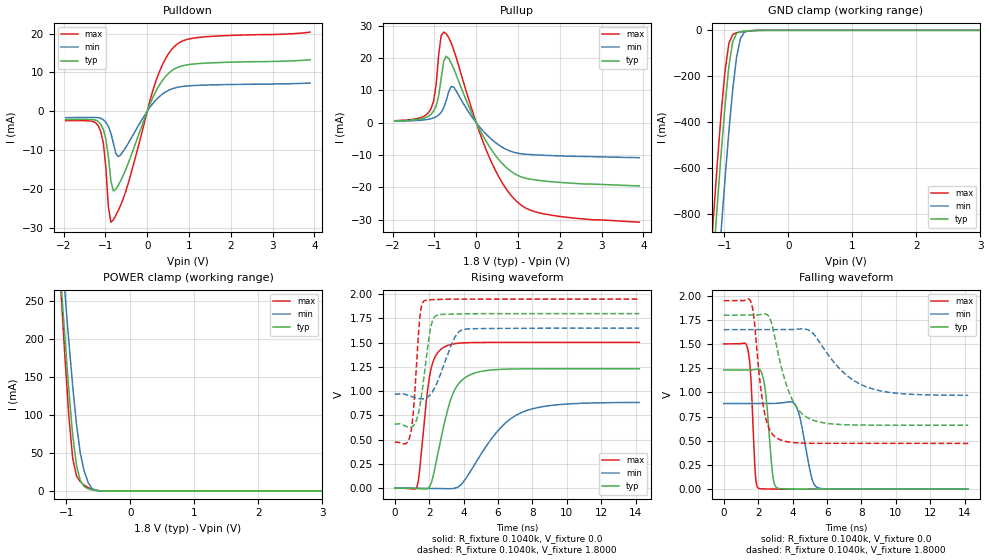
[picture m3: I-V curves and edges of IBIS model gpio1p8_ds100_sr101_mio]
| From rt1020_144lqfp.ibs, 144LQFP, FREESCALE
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[Model] gpio1p8_ds100_sr101_mio
|   Model gpio1p8_ds100_sr101_mio
| This model was characterised for following simulation conditions:
| External (pad) voltage:
|   - Typ: 1.8V,   - Min: 1.65V,   - Max: 1.95V
| Library cells for typ/min/max conditions are connected as defined below:
|  pad - External Pad
|  ipp_do - Core Input
|  ipp_obe - Output Buffer Enable
|  esd_boost - ovdd
|  ipp_dse0 - vssi
|  ipp_dse1 - vssi
|  ipp_dse2 - vddi
|  ipp_fsel0 - vddi
|  ipp_fsel1 - vssi
|  ipp_ina - ipp_ina
|  ipp_ind - ipp_ind
|  ipp_pwr_stable - vddi
|  ipp_sre - vddi
|  ovdd - ovdd
|  ovss - ovss
|  vddi - vddi
|  vssi - vssi
| All other pins connected to ground
Model_type I/O
Polarity   Non-Inverting
Enable   Active-High
Vinl =   0.5400V
Vinh =   1.2600V
Vmeas =  0.9000V
Cref =   0.0F
Rref =   0.1040k
Vref =   0.9000V
C_comp   1.2573pF   1.2208pF   1.3054pF
|C_comp_pullup   0.6439pF   0.6609pF   0.6284pF
|C_comp_pulldown   0.5473pF   0.5786pF   0.5258pF
[Model Spec]
| variable   typ   min   max
Vinh   1.2600V   1.1550V   1.3650V
Vinl   0.5400V   0.4950V   0.5850V
S_overshoot_high   1.8000V   1.6500V   1.9500V
S_overshoot_low   0.0V   0.0V   0.0V
Vmeas   0.9000V   0.8250V   0.9750V
Vref   0.9000V   0.8250V   0.9750V
Cref   0.0F   0.0F   0.0F
Rref   0.1040k   0.1040k   0.1040k
[Temperature Range]   25.0000   0.1050k   -20.0000
[Voltage Range]   1.8000V   1.6500V   1.9500V
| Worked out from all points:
|   slope of the pulldown table from 0 to 0.27 V, typ, clamps not added: 42.3 ohm
|   slope of the pullup table from 0 to 0.27 V, typ, clamps not added: 41.8 ohm
|   GND clamp passes 1 mA (typ) near -0.55 V on its own axis
|   POWER clamp passes 1 mA (typ) near -0.58 V on its own axis
|   rising waveform, R_fixture 0.1040k, V_fixture 0.0: 20-80 % time 1.03ns typ, 2.26ns min, 565ps max; typ from 0 V to 1.23 V
|   rising waveform, R_fixture 0.1040k, V_fixture 1.8000: 20-80 % time 506ps typ, 874ps min, 333ps max; typ from 0.661 V to 1.8 V
|   falling waveform, R_fixture 0.1040k, V_fixture 0.0: 20-80 % time 346ps typ, 561ps min, 230ps max; typ from 1.23 V to 0 V
|   falling waveform, R_fixture 0.1040k, V_fixture 1.8000: 20-80 % time 1.12ns typ, 2.13ns min, 573ps max; typ from 1.8 V to 0.661 V
[Pulldown]
|Voltage   I(typ)   I(min)   I(max)
-1.95V    -2.116mA   -1.648mA   -2.433mA
-1.17V    -2.655mA   -1.64mA    -3.771mA
-1.05V    -4.712mA   -2.199mA   -8.241mA
-990mV    -7.134mA   -2.853mA   -14.49mA
-930mV    -11.63mA   -3.901mA   -24.57mA
-870mV    -17.89mA   -5.605mA   -28.55mA
-810mV    -20.51mA   -8.198mA   -27.94mA
-690mV    -18.99mA   -11.69mA   -25.49mA
210mV     5.219mA    2.926mA    7.83mA
630mV     10.75mA    5.914mA    16.46mA
1.23V     12.27mA    6.677mA    19.01mA
3.9V      13.26mA    7.28mA     20.38mA
[Pullup]
|Voltage   I(typ)   I(min)   I(max)
-1.95V    560uA      440uA      630uA
-1.08V    2.65mA     1.257mA    4.43mA
-960mV    5.224mA    1.847mA    11.81mA
-900mV    8.315mA    2.377mA    20.88mA
-840mV    13.72mA    3.206mA    26.97mA
-780mV    19.01mA    4.561mA    28.05mA
-720mV    20.6mA     6.748mA    27.55mA
-540mV    16.77mA    11mA       22.63mA
240mV     -5.825mA   -3.571mA   -8.452mA
960mV     -16.07mA   -9.337mA   -24.24mA
1.74V     -18.17mA   -10.13mA   -28.48mA
3.9V      -19.55mA   -10.81mA   -30.77mA
[GND_clamp]
|Voltage   I(typ)   I(min)   I(max)
-1.95V    -4.191A    -4.477A    -4.042A
-1.23V    -1.234A    -1.577A    -1.052A
-1.17V    -993.2mA   -1.338A    -811.1mA
-1.11V    -758.1mA   -1.102A    -578.5mA
-1.05V    -533.7mA   -870.8mA   -361.6mA
-990mV    -328mA     -648.8mA   -176.9mA
-930mV    -157.5mA   -441.8mA   -57.56mA
-870mV    -50.13mA   -259.5mA   -18.17mA
-810mV    -13.28mA   -118mA     -10.41mA
-750mV    -5.921mA   -36.52mA   -7.502mA
-630mV    -2.275mA   -2.653mA   -3.283mA
3.9V      0A         0A         0A
[POWER_clamp]
|Voltage   I(typ)   I(min)   I(max)
-1.95V    1.356A     1.328A     1.514A
-1.08V    270.6mA    322.7mA    256.8mA
-1.02V    199mA      258.1mA    173mA
-960mV    131.2mA    195.7mA    97.36mA
-900mV    72.67mA    137.2mA    42.48mA
-840mV    32.99mA    86.34mA    19.5mA
-780mV    13.32mA    48.87mA    11.87mA
-720mV    5.671mA    25.66mA    7.515mA
-660mV    2.793mA    11.19mA    4.477mA
-600mV    1.289mA    3.449mA    2.334mA
-480mV    122.1uA    182.3uA    260.9uA
3.9V      0A         0A         0A
[Ramp]
| variable   typ   min   max
dV/dt_r  0.7391/1.0298n   0.5307/2.2596n   0.9019/0.5652n
dV/dt_f  0.6833/1.1203n   0.4075/2.1341n   0.8860/0.5735n
R_load = 0.1040k
[Rising Waveform]
R_fixture= 0.1040k
V_fixture= 0.0
V_fixture_min= 0.0
V_fixture_max= 0.0
|time   V(typ)   V(min)   V(max)
0s        580.6pV    5.471nV    1.176nV
1.299ns   -3.46mV    257.3uV    24.47mV
1.432ns   -4.528mV   155.2uV    164.2mV
2.064ns   30.64mV    -1.601mV   1.196V
2.798ns   605.7mV    -3.978mV   1.448V
3.567ns   1.042V     4.532mV    1.492V
4.675ns   1.19V      254.8mV    1.502V
6.143ns   1.226V     622.7mV    1.503V
7.696ns   1.231V     803.1mV    1.503V
14.2ns    1.232V     884.6mV    1.503V
[Rising Waveform]
R_fixture= 0.1040k
V_fixture= 1.8000
V_fixture_min= 1.6500
V_fixture_max= 1.9500
|time   V(typ)   V(min)   V(max)
0s        661.1mV    970.1mV    473.3mV
937.6ps   628.9mV    947.4mV    580.8mV
1.103ns   648.4mV    938.3mV    837.9mV
1.438ns   827.4mV    923.7mV    1.728V
1.707ns   1.16V      923.2mV    1.931V
2.11ns    1.674V     975.3mV    1.943V
2.477ns   1.784V     1.097V     1.946V
3.38ns    1.796V     1.516V     1.949V
3.966ns   1.798V     1.635V     1.95V
14.2ns    1.8V       1.65V      1.95V
[Falling Waveform]
R_fixture= 0.1040k
V_fixture= 0.0
V_fixture_min= 0.0
V_fixture_max= 0.0
|time   V(typ)   V(min)   V(max)
0s        1.232V     885.4mV    1.503V
1.379ns   1.232V     885.2mV    1.459V
1.572ns   1.233V     885.2mV    1.154V
1.833ns   1.239V     885.2mV    156mV
2.008ns   1.244V     885.2mV    11.04mV
2.36ns    1.086V     885.2mV    2.499mV
3.101ns   11.96mV    888.5mV    612.3uV
4.249ns   987.7uV    841.8mV    74.66uV
5.465ns   210.9uV    14.34mV    8.599uV
14.2ns    38.11nV    2.863uV    13.42nV
[Falling Waveform]
R_fixture= 0.1040k
V_fixture= 1.8000
V_fixture_min= 1.6500
V_fixture_max= 1.9500
|time   V(typ)   V(min)   V(max)
0s        1.8V       1.65V      1.95V
1.58ns    1.8V       1.65V      1.936V
1.742ns   1.799V     1.65V      1.791V
2.382ns   1.813V     1.65V      776mV
2.747ns   1.736V     1.65V      589.1mV
3.137ns   1.421V     1.65V      522.7mV
4.003ns   915.5mV    1.652V     482.7mV
5.121ns   717.6mV    1.623V     474.3mV
8.143ns   662.5mV    1.069V     473.3mV
14.2ns    661.1mV    970.9mV    473.3mV
